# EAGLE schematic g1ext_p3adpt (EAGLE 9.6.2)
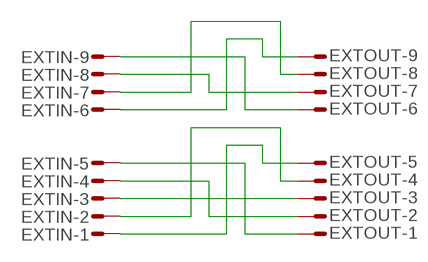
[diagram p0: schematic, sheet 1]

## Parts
EXTIN  M09DS  [M09D]
EXTOUT  M09DS  [M09D]

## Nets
N$1: EXTIN.5 EXTOUT.1
N$2: EXTIN.1 EXTOUT.5
N$3: EXTIN.4 EXTOUT.2
N$4: EXTIN.2 EXTOUT.4
N$5: EXTIN.3 EXTOUT.3
N$6: EXTIN.9 EXTOUT.6
N$7: EXTIN.6 EXTOUT.9
N$8: EXTIN.8 EXTOUT.7
N$9: EXTIN.7 EXTOUT.8

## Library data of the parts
EXTIN EXTOUT = con-subd:M09?S: SUB-D; OC_FARNELL: unknown; OC_NEWARK: unknown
